// TwinCAT 3 PLC project TcComPLCCaller
// ProgramVersion: 3.1.4024.0
// libraries:
//   Tc2_Standard, * (Beckhoff Automation GmbH)
//   Tc2_System, * (Beckhoff Automation GmbH)
//   Tc2_Utilities, * (Beckhoff Automation GmbH)
//   Tc3_Module, * (Beckhoff Automation GmbH)
//   TcComProxyApplication, * (YuYang_Beckhoffsh)
// project tree:
//   / PlcTask.TcTTO
//   POUs/ FB_ProxyPLCCalculationTcComModule.TcPOU, MAIN.TcPOU
// (motion and I/O tree: see PLC project dyntccomproxy)
// real-time tasks:
//   TASK PlcTask: cycle T#10ms, priority 20, ADS port 350
//   TASK PlcTask1: cycle T#10ms, priority 21, ADS port 351
//   TASK PlcTask2: cycle T#10ms, priority 22, ADS port 352
//   TASK PlcTask3: cycle T#10ms, priority 23, ADS port 353
// variable links:
//   TcComPLCCaller/TcComPLCCaller Instance <-> TcComPLCProvider/TcComPLCProvider Instance
//     PlcTask Inputs/MAIN.fbProxyPLCCalculationTcComModule._objectId <-> PlcTask Outputs/MAIN.fbCalc.objID

CONFIGURATION TcComPLCCaller
    RESOURCE PLC ON TwinCAT3
        TASK PlcTask(INTERVAL := T#10ms, PRIORITY := 23);
        PROGRAM MAIN WITH PlcTask : MAIN;
    END_RESOURCE
END_CONFIGURATION

// ---- POUs/MAIN.TcPOU
PROGRAM MAIN
VAR
	
	fbProxyPLCCalculationTcComModule: FB_ProxyPLCCalculationTcComModule;
	
	i 		: INT;	
	a 		: INT := 10;
	b 		: INT := 7;
	nSum 	: INT; // a + b
	nDiff 	: INT; // a - b

	hrCalc 	: HRESULT;

	bInit	: BOOL;
	hr		:HRESULT;
END_VAR

i := i + 1;

IF bInit THEN
	fbProxyPLCCalculationTcComModule.AfterProviderInit(TC_GLOBAL_IID_LIST.IID_I_Calculation);
	bInit:= FALSE;
END_IF

IF fbProxyPLCCalculationTcComModule.ip <> 0 THEN
	fbProxyPLCCalculationTcComModule.Cyclic();
	hrCalc := fbProxyPLCCalculationTcComModule.ip.Addition(a,b,nSum);
	hrCalc := fbProxyPLCCalculationTcComModule.ip.Subtraction(a,b,nDiff);
END_IF

END_PROGRAM

// ---- POUs/FB_ProxyPLCCalculationTcComModule.TcPOU
FUNCTION_BLOCK FB_ProxyPLCCalculationTcComModule EXTENDS FB_ProxyPLCTcComModule
VAR_INPUT
END_VAR
VAR_OUTPUT
END_VAR
VAR
	_iThisProvider		: I_Calculation;
END_VAR

METHOD AfterProviderInit : BOOL
VAR_INPUT
	IID				: IID;
END_VAR


SUPER^.AfterProviderInit(IID:= IID	);

ComQueryInterface(Super^._iProvider,TC_GLOBAL_IID_LIST.IID_I_Calculation ,ADR(_iThisProvider));
END_METHOD

PROPERTY ip : I_Calculation
GET
ip	:= _iThisProvider;
END_GET
END_PROPERTY

END_FUNCTION_BLOCK
